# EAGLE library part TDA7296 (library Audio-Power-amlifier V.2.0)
The TDA7296 is a monolithic integrated circuit in Multiwatt15 package, intended for use as audio class AB amplifier in Hi-Fi field applications (Home Stereo, self powered loudspeakers, Topclass TV). Thanks to the wide voltage range and to the high out current capability it is able to supply the highest power into both 4W and 8W loads even in presence of poor supply regulation, with high Supply Voltage Rejection. The built in muting function with turn on delay simplifies the remote operation avoiding switching on-off noises.
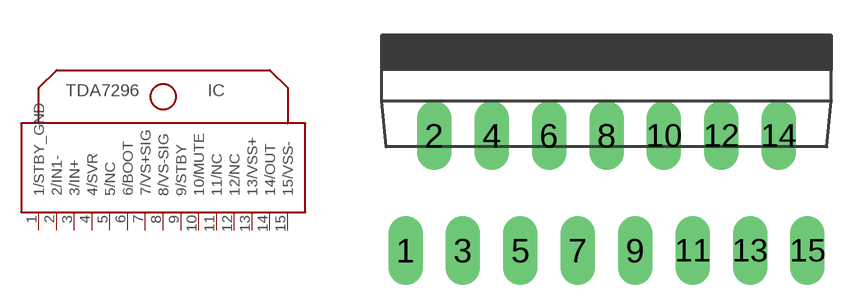
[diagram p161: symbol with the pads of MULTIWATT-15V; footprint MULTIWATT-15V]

Designator prefix IC

## TDA7296  [MULTIWATT-15V]
1  1/STBY_GND
2  2/IN1-  in
3  3/IN+  in
4  4/SVR  in
5  5/NC  nc
6  6/BOOT  in
7  7/VS+SIG  pwr
8  8/VS-SIG  pwr
9  9/STBY  in
10  10/MUTE  in
11  11/NC  nc
12  12/NC  nc
13  13/VSS+  pwr
14  14/OUT  out
15  15/VSS-  pwr

## Footprint MULTIWATT-15V (pad centres in mm)
Multiwatt 15 vertical
drill 1.016 long: 1 -8.89,-5.08; 2 -7.62,0; 3 -6.35,-5.08; 4 -5.08,0; 5 -3.81,-5.08; 6 -2.54,0; 7 -1.27,-5.08; 8 0,0; 9 1.27,-5.08; 10 2.54,0; 11 3.81,-5.08; 12 5.08,0; 13 6.35,-5.08; 14 7.62,0; 15 8.89,-5.08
